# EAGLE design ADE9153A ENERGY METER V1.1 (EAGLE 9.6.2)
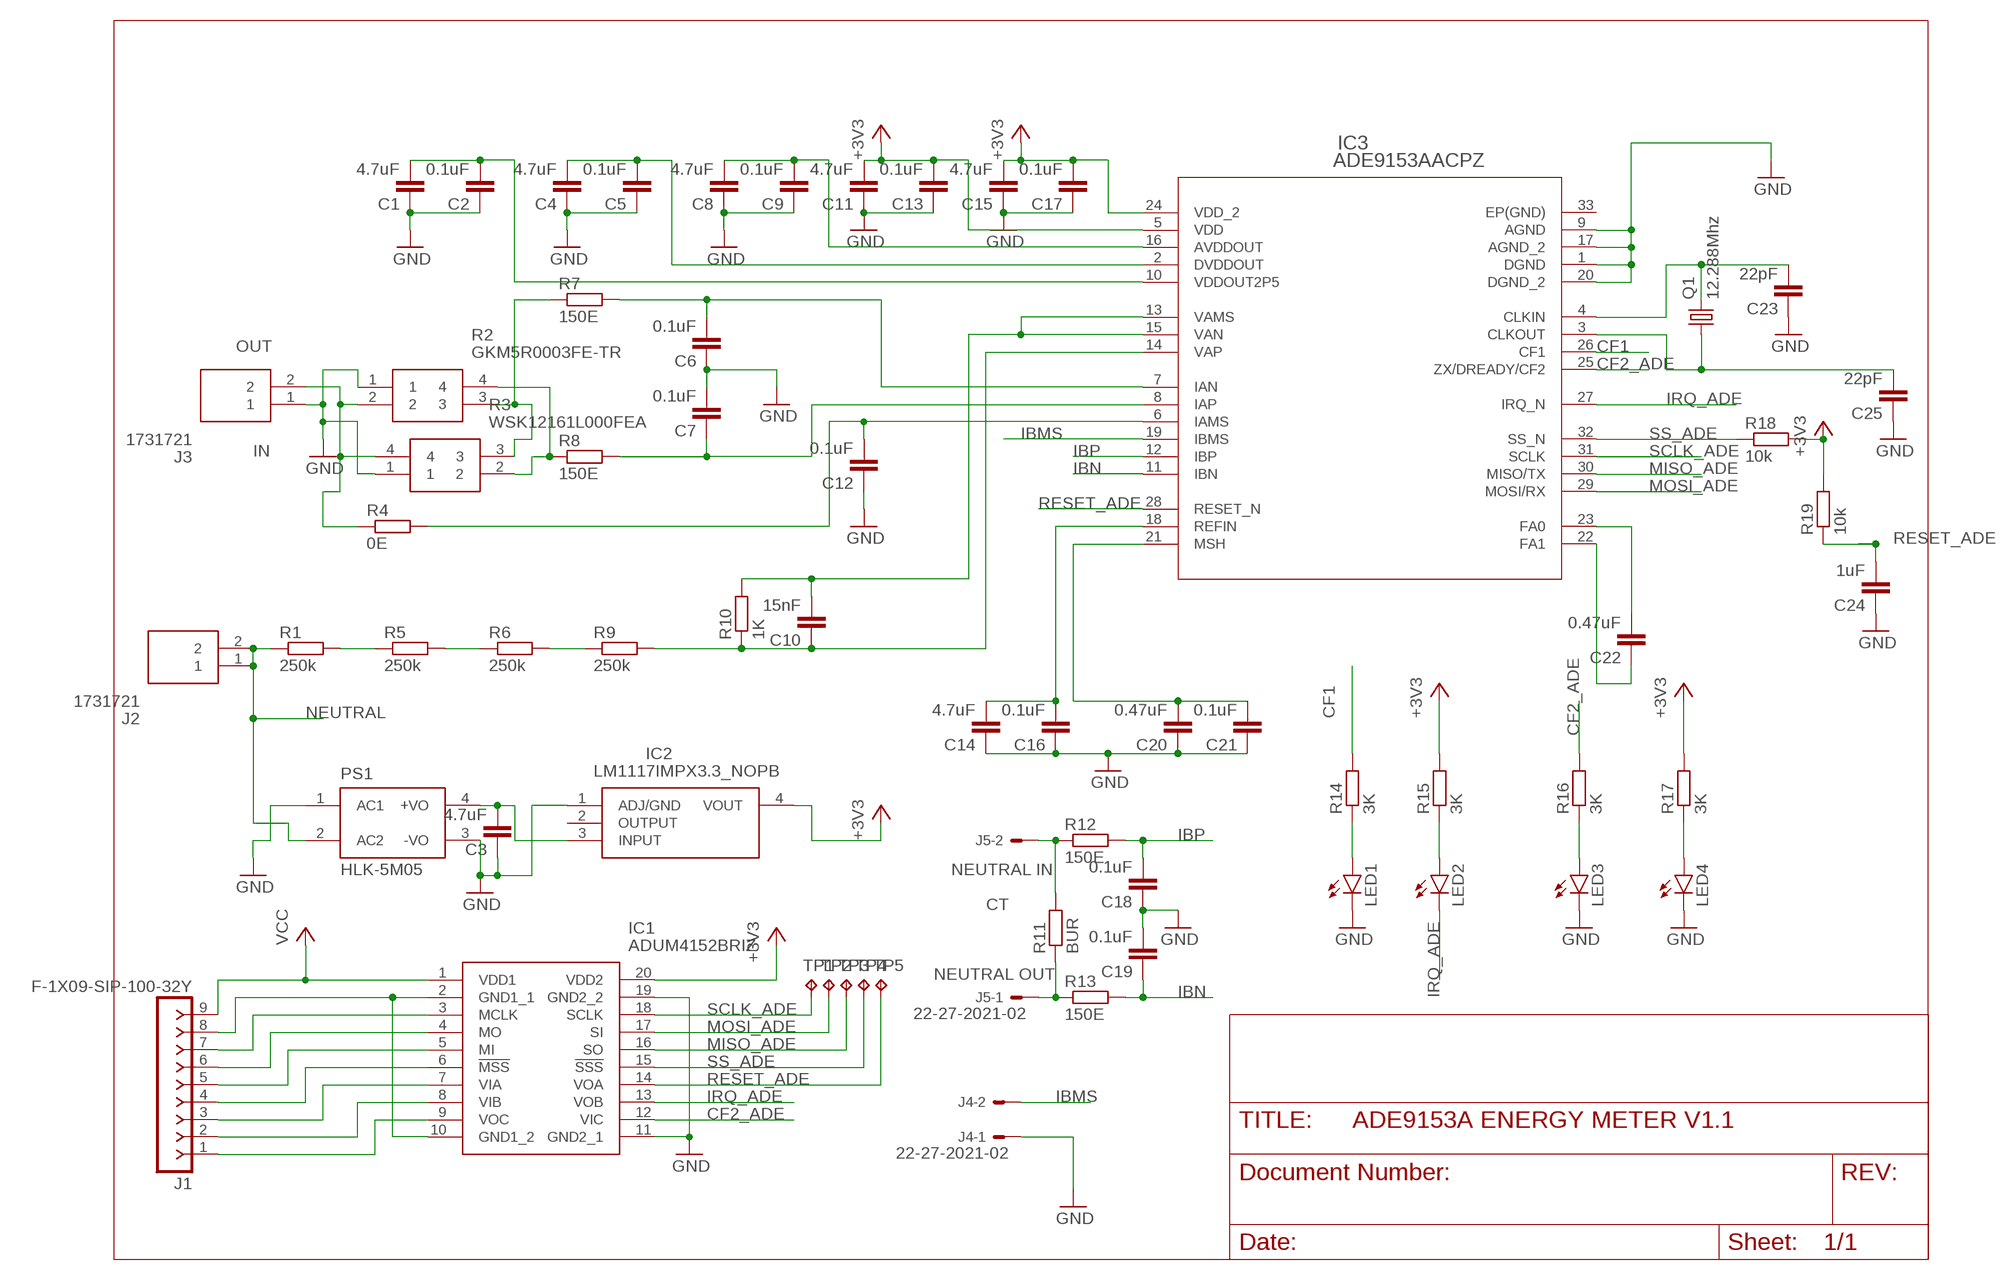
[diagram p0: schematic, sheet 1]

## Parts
C1  4.7uF  C-EUC0805K  [C0805K]
C2  0.1uF  C-EUC0805K  [C0805K]
C3  4.7uF  C-EUC0805K  [C0805K]
C4  4.7uF  C-EUC0805K  [C0805K]
C5  0.1uF  C-EUC0805K  [C0805K]
C6  0.1uF  C-EUC0805K  [C0805K]
C7  0.1uF  C-EUC0805K  [C0805K]
C8  4.7uF  C-EUC0805K  [C0805K]
C9  0.1uF  C-EUC0805K  [C0805K]
C10  15nF  C-EUC0805K  [C0805K]
C11  4.7uF  C-EUC0805K  [C0805K]
C12  0.1uF  C-EUC0805K  [C0805K]
C13  0.1uF  C-EUC0805K  [C0805K]
C14  4.7uF  C-EUC0805K  [C0805K]
C15  4.7uF  C-EUC0805K  [C0805K]
C16  0.1uF  C-EUC0805K  [C0805K]
C17  0.1uF  C-EUC0805K  [C0805K]
C18  0.1uF  C-EUC0805K  [C0805K]
C19  0.1uF  C-EUC0805K  [C0805K]
C20  0.47uF  C-EUC0805K  [C0805K]
C21  0.1uF  C-EUC0805K  [C0805K]
C22  0.47uF  C-EUC0805K  [C0805K]
C23  22pF  C-EUC0805K  [C0805K]
C24  1uF  C-EUC0805K  [C0805K]
C25  22pF  C-EUC0805K  [C0805K]
IC1  ADUM4152BRIZ  [SOIC127P1031X264-20N]
IC2  LM1117IMPX3.3_NOPB  [SOT230P700X180-4N]
IC3  ADE9153AACPZ  [QFN50P500X500X80-33N]
J1  F-1X09-SIP-100-32Y  [SIP-100-09-32Y]
J2  1731721  [1731721]
J3  1731721  [1731721]
J4  22-27-2021-02  [6410-02]
J5  22-27-2021-02  [6410-02]
LED1  LEDCHIPLED_1206  [CHIPLED_1206]
LED2  LEDCHIPLED_1206  [CHIPLED_1206]
LED3  LEDCHIPLED_1206  [CHIPLED_1206]
LED4  LEDCHIPLED_1206  [CHIPLED_1206]
PS1  HLK-5M05  [CONV_HLK-5M05]
Q1  12.288Mhz  CSM-7X-DU  [CSM-7X-DU]
R1  250k  R-EU_R0805  [R0805]
R2  GKM5R0003FE-TR  [GKM5R0003FETR]
R3  WSK12161L000FEA  [WSK12161L000FEA]
R4  0E  R-EU_R0805  [R0805]
R5  250k  R-EU_R0805  [R0805]
R6  250k  R-EU_R0805  [R0805]
R7  150E  R-EU_R0805  [R0805]
R8  150E  R-EU_R0805  [R0805]
R9  250k  R-EU_R0805  [R0805]
R10  1K  R-EU_R0805  [R0805]
R11  BUR  R-EU_R0805  [R0805]
R12  150E  R-EU_R0805  [R0805]
R13  150E  R-EU_R0805  [R0805]
R14  3K  R-EU_R0805  [R0805]
R15  3K  R-EU_R0805  [R0805]
R16  3K  R-EU_R0805  [R0805]
R17  3K  R-EU_R0805  [R0805]
R18  10k  R-EU_R0805  [R0805]
R19  10k  R-EU_R0805  [R0805]
TP1  TPTP10R  [TP10R]
TP2  TPTP10R  [TP10R]
TP3  TPTP10R  [TP10R]
TP4  TPTP10R  [TP10R]
TP5  TPTP10R  [TP10R]

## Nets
+3V3: C11.2 C13.2 C15.2 C17.2 IC1.20(VDD2) IC2.4(VOUT) IC3.5(VDD) IC3.24(VDD_2) R15.2 R17.2 R18.2 R19.2
CF1: IC3.26(CF1) R14.2
CF2_ADE: IC1.12(VIC) IC3.25(ZX/DREADY/CF2) R16.2
GND: C1.1 C2.1 C3.1 C4.1 C5.1 C6.1 C7.2 C8.1 C9.1 C11.1 C12.1 C13.1 C14.1 C15.1 C16.1 C17.1 C18.1 C19.2 C20.1 C21.1 C23.1 C24.1 C25.1 IC1.11(GND2_1) IC1.19(GND2_2) IC2.1(ADJ/GND) IC3.1(DGND) IC3.9(AGND) IC3.17(AGND_2) IC3.20(DGND_2) J3.1 J4.1 LED1.C LED3.C LED4.C PS1.1(AC1) PS1.3(-VO) R2.1 R3.1
IBMS: IC3.19(IBMS) J4.2
IBN: C19.1 IC3.11(IBN) R13.2
IBP: C18.2 IC3.12(IBP) R12.2
IRQ_ADE: IC1.13(VOB) IC3.27(IRQ_N) LED2.C
MISO_ADE: IC1.16(SO) IC3.30(MISO/TX) TP3.TP
MOSI_ADE: IC1.17(SI) IC3.29(MOSI/RX) TP2.TP
N$1: R2.4 R3.2 R8.1
N$2: R2.3 R3.3 R7.1
N$3: J5.2 R11.2 R12.1
N$4: C6.2 IC3.7(IAN) R7.2
N$5: C7.1 IC3.8(IAP) R8.2
N$6: C12.2 IC3.6(IAMS) R4.2
N$7: C3.2 IC2.3(INPUT) PS1.4(+VO)
N$8: R1.2 R5.1
N$9: R5.2 R6.1
N$10: R6.2 R9.1
N$11: C10.1 IC3.14(VAP) R9.2 R10.1
N$12: C10.2 IC3.13(VAMS) IC3.15(VAN) R10.2
N$13: C8.2 C9.2 IC3.16(AVDDOUT)
N$14: C14.2 C16.2 IC3.18(REFIN)
N$15: LED1.A R14.1
N$16: LED2.A R15.1
N$17: C1.2 C2.2 IC3.10(VDDOUT2P5)
N$18: C4.2 C5.2 IC3.2(DVDDOUT)
N$19: C23.2 IC3.4(CLKIN) Q1.2
N$20: C25.2 IC3.3(CLKOUT) Q1.1
N$22: C22.2 IC3.23(FA0)
N$23: C22.1 IC3.22(FA1)
N$24: IC1.2(GND1_1) IC1.10(GND1_2) J1.8
N$25: C20.2 C21.2 IC3.21(MSH)
N$26: IC1.3(MCLK) J1.7
N$27: IC1.4(MO) J1.6
N$28: IC1.5(MI) J1.5
N$29: IC1.6(!MSS) J1.4
N$30: IC1.7(VIA) J1.3
N$31: IC1.8(VIB) J1.2
N$32: IC1.9(VOC) J1.1
N$33: LED3.A R16.1
N$34: LED4.A R17.1
N$35: J5.1 R11.1 R13.1
N$38: J3.2 R2.2 R3.4 R4.1
NEUTRAL: J2.1 J2.2 PS1.2(AC2) R1.1
RESET_ADE: C24.2 IC1.14(VOA) IC3.28(RESET_N) R19.1 TP5.TP
SCLK_ADE: IC1.18(SCLK) IC3.31(SCLK) TP1.TP
SS_ADE: IC1.15(!SSS) IC3.32(SS_N) R18.1 TP4.TP
VCC: IC1.1(VDD1) J1.9
Unconnected: IC2.2(OUTPUT) IC3.33(EP(GND))

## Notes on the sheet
- OUT
- IN
- NEUTRAL IN
- CT
- NEUTRAL OUT

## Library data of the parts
C1-C25 = rcl:C-EU: CAPACITOR, European symbol; SPICEPREFIX: C
IC1 = IC:ADUM4152BRIZ: Analog Devices ADUM4152BRIZ PCB SMT, 7-channel Digital Isolator for SPI 34MBps, 5 kV ac, 20-Pin SOIC Source: Datasheet; ARROW_PART_NUMBER: ADUM4152BRIZ; ARROW_PRICE-STOCK: https://www.arrow.com/en/products/adum4152briz/analog-devices; DESCRIPTION: Analog Devices ADUM4152BRIZ PCB SMT, 7-channel Digital Isolator for SPI 34MBps, 5 kV ac, 20-Pin SOIC; HEIGHT: 2.64mm; MANUFACTURER_NAME: Analog Devices; MANUFACTURER_PART_NUMBER: ADUM4152BRIZ; MOUSER_PART_NUMBER: 584-ADUM4152BRIZ; MOUSER_PRICE-STOCK: https://www.mouser.co.uk/ProductDetail/Analog-Devices/ADUM4152BRIZ/?qs=iCT64eccu7h2dAwNIWQgpQ%3D%3D
IC2 = IC:LM1117IMPX3.3_NOPB: Space Saving 800mA Low-Dropout Linear Regulator with Internal Current Limit 4-SOT-223 -40 to 125 Source: Datasheet; DESCRIPTION: Space Saving 800mA Low-Dropout Linear Regulator with Internal Current Limit 4-SOT-223 -40 to 125; HEIGHT: 1.8mm; MANUFACTURER_NAME: Texas Instruments; MANUFACTURER_PART_NUMBER: LM1117IMPX3.3/NOPB
IC3 = ADE9153AACPZ:ADE9153AACPZ; AVAILABILITY: Unavailable; DESCRIPTION: Single Phase Meter IC 32-LFCSP (5x5); MF: Analog Devices; MP: ADE9153AACPZ; PACKAGE: LFCSP -32 Analog Devices; PRICE: None
J1 = con-headers-jp:F-1X09-: FEMALE HEADER
J2 J3 = IC:1731721: 2 way PCB mount screw terminal,7.62mm 2 way PCB mount screw terminal,7.62mm; ARROW_PART_NUMBER: 1731721; ARROW_PRICE-STOCK: https://www.arrow.com/en/products/1731721/phoenix-contact; DESCRIPTION: 2 way PCB mount screw terminal,7.62mm 2 way PCB mount screw terminal,7.62mm; HEIGHT: mm; MANUFACTURER_NAME: Phoenix Contact; MANUFACTURER_PART_NUMBER: 1731721; MOUSER_PART_NUMBER: 651-1731721; MOUSER_PRICE-STOCK: https://www.mouser.co.uk/ProductDetail/Phoenix-Contact/1731721?qs=Hp4IEBVVqKLHS2iTGzgL4g%3D%3D
J4 J5 = con-molex:22-?-02: CONNECTOR; MF: MOLEX; OC_FARNELL: unknown; OC_NEWARK: unknown
LED1-LED4 = led:LED: LED
PS1 = HLK-5M05:HLK-5M05: AC DC 220V to 5V 5W 5Watt Isolated Switching Step-Down Power Supply Module Converter; AVAILABILITY: Unavailable; MF: Hi-link; MP: HLK-5M05; PACKAGE: Package; PRICE: None
Q1 = crystal:CSM-7X-DU: SMD CRYSTAL; OC_FARNELL: unknown; OC_NEWARK: unknown
R1 R4-R19 = rcl:R-EU_: RESISTOR, European symbol; SPICEPREFIX: R
R2 = IC:GKM5R0003FE-TR: FK/GK Series Metal Alloy Low-Resistance Chip Resistor Source: Datasheet; DESCRIPTION: FK/GK Series Metal Alloy Low-Resistance Chip Resistor; HEIGHT: 3.5mm; MANUFACTURER_NAME: Ohmite; MANUFACTURER_PART_NUMBER: GKM5R0003FE-TR; MOUSER_PART_NUMBER: 588-GKM5R0003FE-TR; MOUSER_PRICE-STOCK: https://www.mouser.co.uk/ProductDetail/Ohmite/GKM5R0003FE-TR/?qs=0lSvoLzn4L%252BprfgVSUIuyQ%3D%3D
R3 = WSK12161L000FEA:WSK12161L000FEA: Check prices; AVAILABILITY: Warning; DESCRIPTION: 1 mOhms ±1% 3W Chip Resistor Wide 1612 (3831 Metric), 1216 Current Sense, Moisture Resistant, Pulse Withstanding Metal Element; MF: Vishay Dale; MP: WSK12161L000FEA; PACKAGE: 1216 Vishay Dale; PRICE: None; PURCHASE-URL: https://pricing.snapeda.com/search/part/WSK12161L000FEA/?ref=eda
TP1-TP5 = testpad:TP: Test pad

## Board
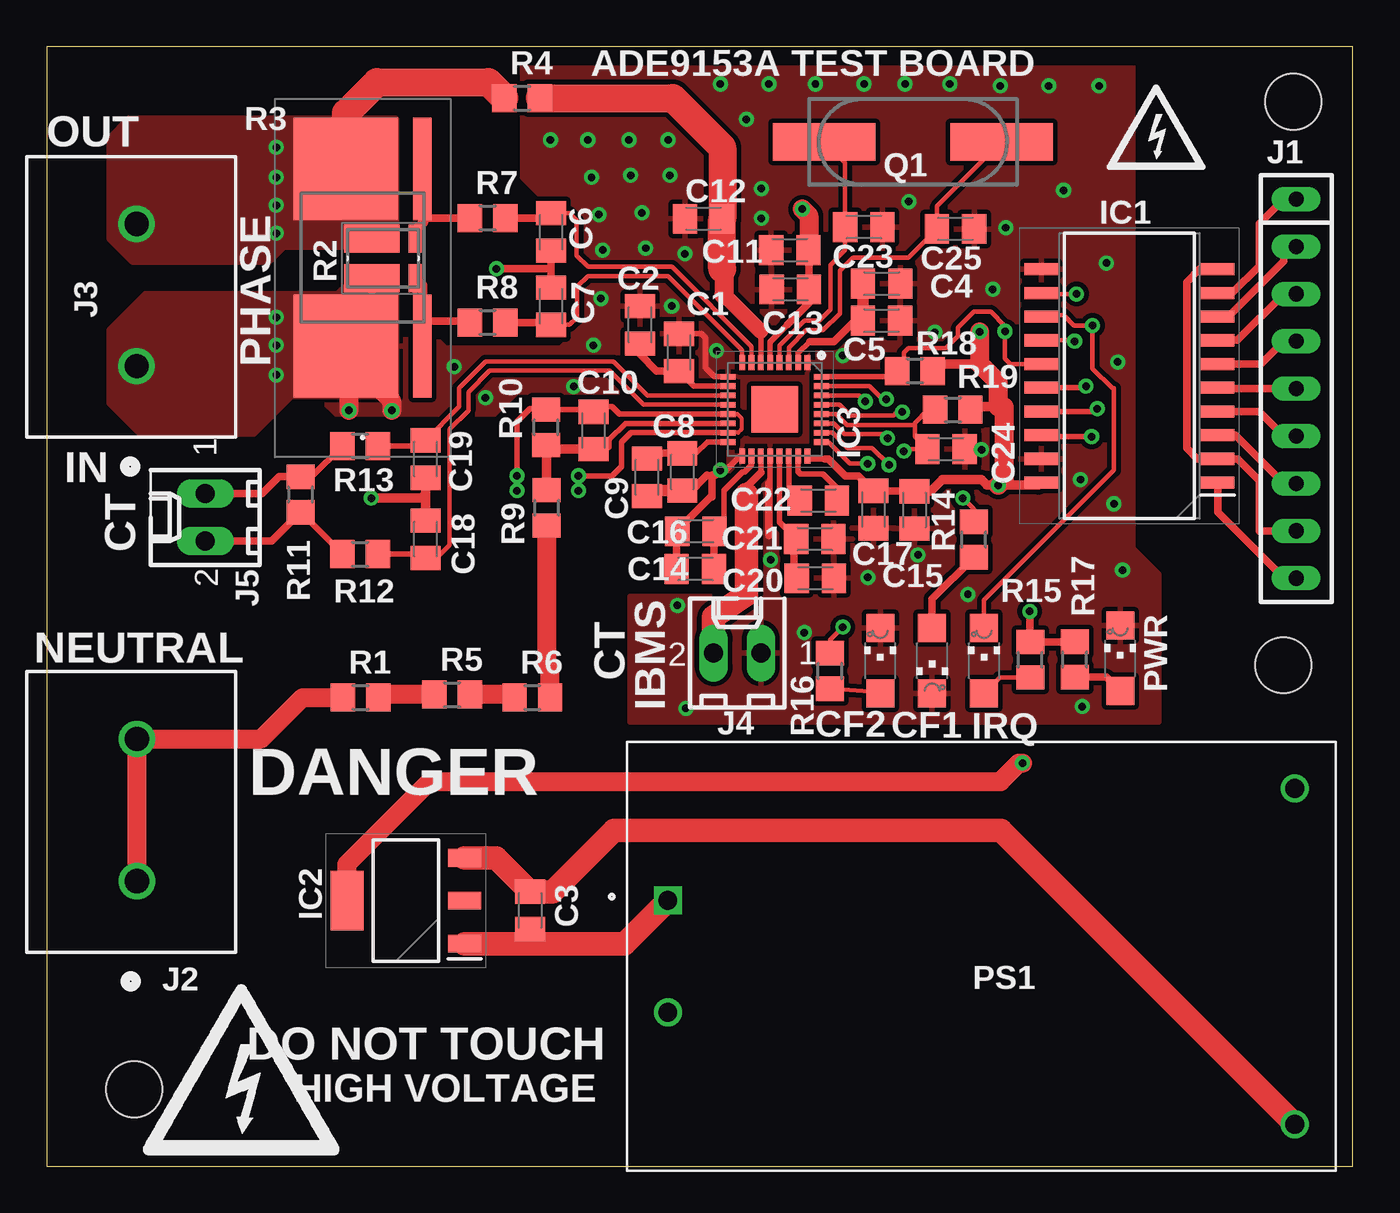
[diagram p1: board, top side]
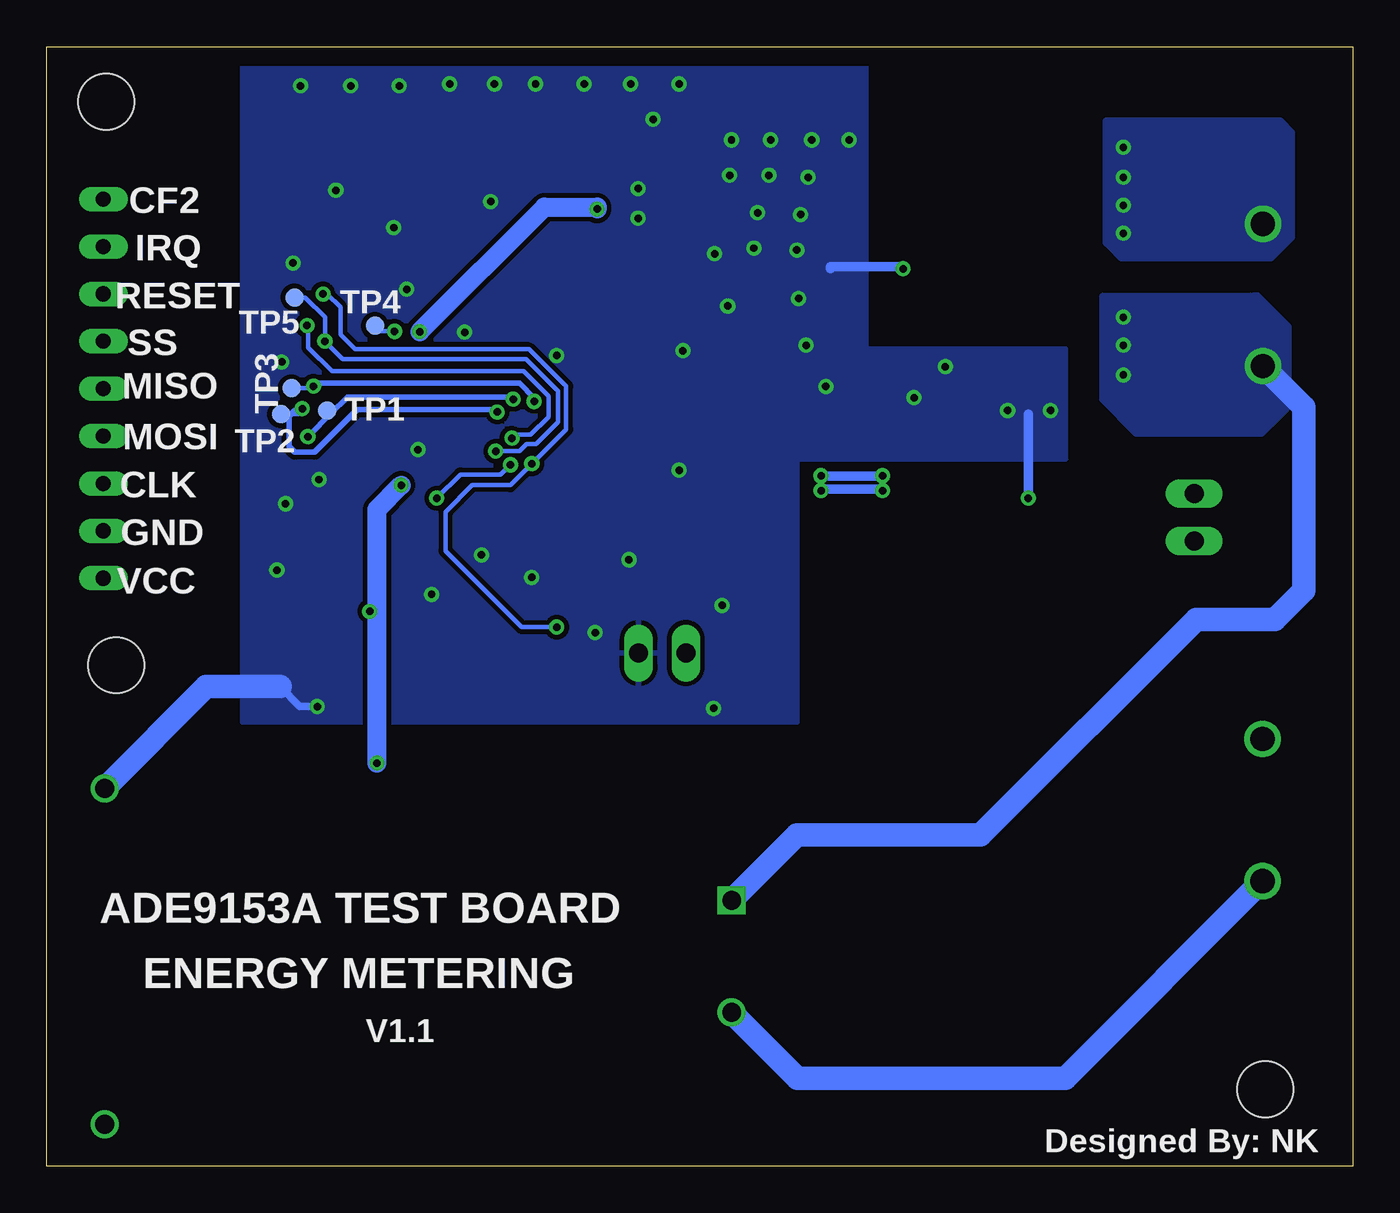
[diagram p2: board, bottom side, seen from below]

Size 70 x 60 mm. Coordinates in mm from the lower left corner, seen from the top.
Outline: 0,0 70,0 70,60 0,60 0,0
Copper layers (1*16): Top 0.035mm / dielectric 1.5mm / Bottom 0.035mm
Design rules "default": minimum track width 6mil, minimum drill 0.35mm, track to track 6mil, track to pad 6mil, pad to pad 6mil, via to via 6mil, smd to smd 6mil, copper to edge 40mil, drill to drill 6mil, minimum pad ring 10mil, minimum via ring 8mil, stop-mask expansion 4mil, vias tented up to drill 0mil, thermal gap 10mil
Holes 3 mm at 4.69,4.13 66.8,57.04 66.27,26.85

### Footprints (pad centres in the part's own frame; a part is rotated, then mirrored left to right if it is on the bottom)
C0805K = smd 1.3 x 1.6: 1 -1,0; 2 1,0
SOIC127P1031X264-20N = smd 1.8 x 0.65: 1 -4.725,5.715; 2 -4.725,4.445; 3 -4.725,3.175; 4 -4.725,1.905; 5 -4.725,0.635; 6 -4.725,-0.635; 7 -4.725,-1.905; 8 -4.725,-3.175; 9 -4.725,-4.445; 10 -4.725,-5.715; 11 4.725,-5.715; 12 4.725,-4.445; 13 4.725,-3.175; 14 4.725,-1.905; 15 4.725,-0.635; 16 4.725,0.635; 17 4.725,1.905; 18 4.725,3.175; 19 4.725,4.445; 20 4.725,5.715
SOT230P700X180-4N = smd 1.75 x 0.95: 1 -3.15,2.3; 2 -3.15,0; 3 -3.15,-2.3 | smd 1.75 x 3.2: 4 3.15,0
QFN50P500X500X80-33N = smd 0.8 x 0.3: 1 -2.5,1.75; 2 -2.5,1.25; 3 -2.5,0.75; 4 -2.5,0.25; 5 -2.5,-0.25; 6 -2.5,-0.75; 7 -2.5,-1.25; 8 -2.5,-1.75; 17 2.5,-1.75; 18 2.5,-1.25; 19 2.5,-0.75; 20 2.5,-0.25; 21 2.5,0.25; 22 2.5,0.75; 23 2.5,1.25; 24 2.5,1.75 | smd 0.3 x 0.8: 9 -1.75,-2.5; 10 -1.25,-2.5; 11 -0.75,-2.5; 12 -0.25,-2.5; 13 0.25,-2.5; 14 0.75,-2.5; 15 1.25,-2.5; 16 1.75,-2.5; 25 1.75,2.5; 26 1.25,2.5; 27 0.75,2.5; 28 0.25,2.5; 29 -0.25,2.5; 30 -0.75,2.5; 31 -1.25,2.5; 32 -1.75,2.5 | smd 2.5 x 2.5: 33 0,0
SIP-100-09-32Y = drill 0.813 long: 1 -10.16,0; 2 -7.62,0; 3 -5.08,0; 4 -2.54,0; 5 0,0; 6 2.54,0; 7 5.08,0; 8 7.62,0; 9 10.16,0
1731721 = drill 1.3 pad 1.95: 1 -3.92,-0.11; 2 3.7,-0.11
6410-02 = drill 1.016 long: 1 1.27,0; 2 -1.27,0
CHIPLED_1206 = smd 1.5 x 1.5: A 0,-1.75; C 0,1.75
CONV_HLK-5M05 = drill 1 pad 1.5 square: 1 -16.8,3 | drill 1 pad 1.5: 2 -16.8,-3; 3 16.8,9; 4 16.8,-9
CSM-7X-DU = smd 5.5 x 2: 1 -4.75,0; 2 4.75,0
R0805 = smd 1.3 x 1.5: 1 -0.95,0; 2 0.95,0
GKM5R0003FETR = smd 5.5 x 5.6: 1 -4.75,0.9; 2 4.75,0.9 | smd 5.5 x 1: 3 4.75,-3.2; 4 -4.75,-3.2
WSK12161L000FEA = smd 2.95 x 1.495: 1 -0.6,-1.053; 4 -0.6,1.053 | smd 0.7 x 1.495: 2 1.725,-1.053; 3 1.725,1.053
TP10R = smd 1 x 1: TP 0,0

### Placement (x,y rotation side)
C1  33.89,43.61 270 top
C2  31.79,45.09 270 top
C3  25.91,13.71 90 top
C4  44.75,47.29 180 top
C5  44.74,45.31 180 top
C6  27.03,50.07 90 top
C7  27.03,46.09 90 top
C8  34.06,37.21 90 top
C9  32.17,36.92 90 top
C10  29.31,39.43 90 top
C11  39.83,49.09 0 top
C12  35.21,50.77 0 top
C13  39.85,46.99 0 top
C14  34.76,32.01 0 top
C15  46.51,35.17 90 top
C16  34.79,34.03 0 top
C17  44.31,35.19 90 top
C18  20.3,33.6 270 top
C19  20.3,37.9 270 top
C20  41.19,31.51 180 top
C21  41.17,33.61 180 top
C22  41.35,35.67 0 top
C23  43.79,50.33 180 top
C24  48.2,38.43 180 top
C25  48.71,50.23 180 top
IC1  58.02,42.35 180 top
IC2  19.25,14.23 180 top
IC3  39.02,40.56 270 top
J1  66.96,41.67 270 top
J2  4.73,19.2 90 top
J3  4.71,46.8 90 top
J4  37.01,27.5 0 top
J5  8.5,34.77 90 top
LED1  47.45,27.09 180 top
LED2  50.23,27.09 0 top
LED3  44.67,27.09 0 top
LED4  57.53,27.22 0 top
PS1  50.09,11.25 0 top
Q1  46.42,54.9 180 top
R1  16.83,25.12 0 top
R2  16.94,48.7 90 top
R3  18.03,48.65 0 top
R4  25.48,57.24 0 top
R5  21.73,25.27 0 top
R6  26.03,25.12 0 top
R7  23.63,50.82 0 top
R8  23.63,45.22 0 top
R9  26.8,35.29 90 top
R10  26.76,39.6 90 top
R11  13.6,36 270 top
R12  16.8,32.8 0 top
R13  16.8,38.6 0 top
R14  49.68,33.58 90 top
R15  52.71,27.14 90 top
R16  41.98,26.54 90 top
R17  55.09,27.16 90 top
R18  46.53,42.62 0 top
R19  48.56,40.54 0 top
TP1  54.97,40.5 0 bottom
TP2  57.44,40.3 0 bottom
TP3  56.88,41.69 0 bottom
TP4  52.4,45.05 0 bottom
TP5  56.72,46.56 0 bottom

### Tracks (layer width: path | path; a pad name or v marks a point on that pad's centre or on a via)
+3V3  (via drill 0.4)
  Top 0.305: IC3.5 38.77,44.17 39.7,45.1 | 40.85,49.07 C11.2 | IC3.24 40.93,37.9 41.7,37.9
  Top 0.406: 39.7,45.1 40.85,46.25 C13.2 40.85,49.07 | 41.7,37.9 41.9,37.9 42.8,37 43.5,37 C17.2 46.49,36.19 C15.2 | R17.2 55.09,28.36 54.83,28.09 R15.2 52.69,28.21 v52.69,29.73
  Top 0.508: R18.2 47.86,43 50,43 | R19.2 49.67,40.7 51,40.7 51.3,40.7 | IC1.20 53.16,36.5 v51,36.5 50.4,36.5 50.1,36.8 48,36.8 47.39,36.19 46.49,36.19
  Top 1.016: IC2.4 16.1,16.2 20.52,20.62 51.12,20.62 52.1,21.6 v52.3,21.6 | v51,36.5 51.3,36.8 51.3,40.7 | 51,40.7 51,42 50.01,42.99 | 50.01,42.99 50,43 | 50.01,42.99 v50.01,44.72 | v40.5,51.3 40.85,50.95 40.85,49.07
  Bottom 0.406: v52.69,29.73 52.3,30.12
  Bottom 1.016: v52.3,21.6 52.3,30.12 52.3,35.2 v51,36.5 | v50.01,44.72 43.33,51.4 40.5,51.4 v40.5,51.3
CF1  (via drill 0.4)
  Top 0.254: IC3.26 42.12,39.31 42.92,38.5 44.24,38.5 v45.15,37.59 | v49.1,35.8 49.68,35.22 R14.2
  Bottom 0.254: v45.15,37.59 45.67,37.07 47.83,37.07 v49.1,35.8
CF2_ADE  (via drill 0.4)
  Top 0.254: IC3.25 41.89,38.81 43.05,37.65 v44,37.65 | v42.67,28.89 41.98,28.2 R16.2 | v55.19,46.74 53.36,46.74 IC1.12
  Bottom 0.254: v42.67,28.89 44.54,28.89 48.63,32.98 48.63,35.07 47.2,36.5 45.15,36.5 v44,37.65 42.16,39.49 42.16,41.8 44.15,43.79 53.47,43.79 54.25,44.57 54.25,46.03 54.96,46.74 v55.19,46.74
GND  (via drill 0.4)
  Top 0.254: 38.77,36.67 38.7,36.6
  Top 0.305: IC3.20 38.77,36.67 | IC3.17 37.16,38.06 36.14,37.04 35.66,37.04 35.65,37.04 35.4,37.04 | 34.31,35.95 C8.1 | IC3.9 35.79,42.31 35.3,42.8 35.3,44.4 35.09,44.61 C1.1
  Top 0.406: C7.2 27.03,48.1 | 27.03,48.1 C6.1 | 27.03,48.1 v24.1,48.1 | 34.31,35.95 35.4,37.04 | R3.1 17.43,45.02 16.2,43.79 | 38.7,36.6 38.7,33.8 | 35.66,37.04 35.66,35.85 35.58,35.85 33.79,34.06 | C16.1 33.79,34.06 | v36.1,37.3 35.84,37.04 35.65,37.04 | C14.1 33.76,34.03 33.79,34.06
  Top 0.508: C18.1 20.3,36 | 20.3,36 C19.2 | 20.3,36 20.1,35.8 v17.4,35.8 | C24.1 50.07,38.43 v50.1,38.4
  Top 0.61: C8.1 32.46,36.21 C9.1
  Top 1.016: v16.2,40.5 16.2,43.79 R2.1 16.04,43.46 18.5,41 v18.5,40.5
  Top 1.27: IC2.1 26.1,11.93 | C3.1 26.1,12.52 26.1,11.93 | PS1.1 30.97,11.93 26.1,11.93
  Bottom 0.406: v55.5,24.63 56.43,24.63 57.5,25.7
  Bottom 0.508: v24.1,48.1 24.2,48.2 28,48.2 28,48.1 | v17.4,35.8 17.4,40.3
  Bottom 1.27: PS1.3 61.44,25.7 57.5,25.7 | J3.1 2.62,40.68 2.62,30.86 4.18,29.3 8.4,29.3 19.95,17.75 29.79,17.75 PS1.1
  other vias: 27,55 29,55 31.2,55 33.3,55 33.4,53.1 31.3,53.1 29.2,53 29.6,51 31.9,51.1 29.8,49.1 34.2,48.9 32.1,49.2 29.7,46.5 29.3,44 21.84,42.85 12.3,45.5 12.3,44 12.3,42.4 35.9,43.7 42.67,43.45 40.6,28.6 44.01,31.56 46.7,32.76 49.37,30.64 57.66,31.94 55.4,36.8 57.2,35.5 57.4,43.1 50.7,47 47.6,44.7 54.5,52.3 56.4,57.9 38.7,58 36.1,58 41.2,58 43.8,58 46,58 48.4,58 51.1,57.9 53.7,57.9 37.5,56.1 38.3,52.4 46.2,51.7 51.4,50.3 56.8,48.4 38.3,50.8 33.5,46.1 34.26,24.54 38.8,32.5 23.52,41.18 28.24,41.79 33.8,30.06
  pour Top (isolate 0.254): 25.5,59.2 25.5,53 28.2,50.3 28.2,44.5 27.55,43.85 21.35,43.85 20.9,44.3 15.6,44.3 14.8,43.5 14.8,41 15.5,40.3 24,40.3 25.2,41.5 35.4,41.5 36.58,40.32 36.58,30.52 31.26,30.52 31.26,23.82 59.6,23.82 59.6,31.7 58.2,33.1 58.2,60.8 25.5,60.8 25.5,59.3 25.6,59.2
  pour Bottom (isolate 0.254): 15.4,37.9 29.8,37.9 29.8,23.8 59.5,23.8 59.5,60.7 26.4,60.7 26.1,60.4 26.1,43.8 15.4,43.8
  pour Top (no thermals): 16.2,47.9 16.2,47.3 15.6,46.7 5.3,46.7 3.4,44.8 3.4,40.9 5,39.3 11.1,39.3 13.1,41.3 18.6,41.3 18.7,41.4 18.7,47.9
  pour Bottom (no thermals): 5.2,46.7 3.5,45 3.5,40.7 4.9,39.3 11.6,39.3 13.4,41.1 13.4,46.6 5.3,46.6
IBMS
  Top 0.305: IC3.19 38.27,37.17
  Top 0.406: 38.27,37.17 37.5,36.4
  Top 0.508: 37.5,36.4 37.5,36
  Top 1.27: 37.5,36 37.5,30.63 35.74,29.42 J4.2
IBN
  Top 0.254: C19.1 22.1,40.7 22.1,41.7 23.51,43.11 30.39,43.11 32.19,41.31 IC3.11
  Top 0.305: C19.1 20,38.6 R13.2
IBP
  Top 0.254: IC3.12 31.99,40.81 30.17,42.63 23.73,42.63 22.6,41.5 22.6,40.5 21.6,39.5 21.6,33.3 20.9,32.6 C18.2
  Top 0.305: R12.2 20.1,32.8 C18.2
IRQ_ADE  (via drill 0.4)
  Top 0.254: IC3.27 42.19,39.81 42.76,39.24 44.76,39.24 44.98,39.02 v45.06,39.02 | IC1.13 53.37,45.6 54.5,45.6 55.04,45.06 v56.04,45.06 56.04,42.76 57.1,41.7 57.2,41.7 57.2,37.3 50.23,30.33 LED2.C
  Bottom 0.254: v45.06,39.02 44.87,39.21 44.06,39.21 43.11,40.16 43.11,41.27 44.44,42.6 54.7,42.6 55.98,43.88 55.98,44.99 v56.04,45.06
MISO_ADE  (via drill 0.4)
  Top 0.254: IC3.30 43.55,41.31 v43.87,40.99
  Top 0.305: v55.7,41.8 55.62,41.72 IC1.16
  Bottom 0.254: TP3.TP 55.81,41.69 v55.7,41.8
  Bottom 0.305: v43.87,40.99 43.87,41.17 44.66,41.96 55.54,41.96 v55.7,41.8
MOSI_ADE  (via drill 0.4)
  Top 0.254: IC3.29 42.49,40.81 43.07,40.23 45.38,40.23 45.57,40.42 v45.85,40.42
  Top 0.305: v56.3,40.6 56.15,40.45 IC1.17
  Bottom 0.254: TP2.TP 56.5,40.3 56.3,40.5
  Bottom 0.305: v45.85,40.42 45.98,40.55 53.35,40.55 55.63,38.27 56.7,38.27 57,38.57 57,40.2 56.7,40.5 56.3,40.5 v56.3,40.6
N$1
  Top 0.254: 20.53,45.3 19.75,46.08 R3.2 | 22.68,45.3 R8.1
  Top 0.406: 20.53,45.3 22.68,45.3
  Top 0.508: R2.4 20.14,47.21 R3.2
N$2
  Top 0.254: R2.3 20.14,50.8 | 22.66,50.8 R7.1
  Top 0.406: 20.14,50.8 22.66,50.8
  Top 0.508: R3.3 19.75,50.16 20.2,50.6 20.2,53.39 R2.3
N$3
  Top 0.305: R12.1 R11.2
  Top 0.406: J5.2 12.05,33.5 R11.2
N$4
  Top 0.254: 26.91,50.95 C6.2 | 26.78,50.82 C6.2 | C6.2 28.03,51.07 28.4,50.7 28.4,48.8 29,48.2 33.5,48.2 37.77,43.93 IC3.7
  Top 0.406: R7.2 26.78,50.82
N$5
  Top 0.254: 26.9,45.22 C7.1 28.03,45.09 28.43,45.49 28.43,47.13 29,47.7 33.3,47.7 37.27,43.73 IC3.8
  Top 0.406: R8.2 26.9,45.22
N$6
  Top 0.305: IC3.6 38.27,44.73
  Top 0.813: 38.27,44.73 36.3,46.7
  Top 1.016: 36.2,48.1 36.3,48 36.3,46.7
  Top 1.5: R4.2 33.56,57.24 36.21,54.59 C12.2 36.2,50.76 36.2,48.1
N$7
  Top 1.27: IC2.3 24.09,16.53 C3.2 27.12,14.71 30.41,18 51.14,18 PS1.4
N$8
  Top 1.016: R1.2 17.93,25.27 R5.1
N$9
  Top 1.016: R5.2 24.93,25.27 R6.1
N$10
  Top 1.016: R9.1 26.8,27 26.98,26.82 R6.2
N$11
  Top 0.305: IC3.14 31.01,39.81 30.13,38.93 30.13,38.55 30.01,38.43 C10.1
  Top 0.508: R9.2 26.8,38.61 | 26.8,38.61 R10.1 | C10.1 26.98,38.43 26.8,38.61
N$12  (via drill 0.4)
  Top 0.203: IC3.13 37.02,40.31 37.23,40.1 37.23,39.49 37.05,39.31 IC3.15
  Top 0.305: IC3.15 31.31,39.31 30.8,38.8 30.8,37.5 30.3,37 28.6,37 | v28.5,36.2 28.5,36.9 28.6,37 | 28.6,37 v28.5,37 | 29.19,40.55 R10.2 26.71,40.6 25.9,40.6 25.2,39.9 v25.2,37 v25.2,36.2 | 29.19,40.55 C10.2 | IC3.13 30.69,40.31 30.3,40.7 29.34,40.7 29.19,40.55
  Bottom 0.305: v28.5,37 v28.5,36.2 | v25.2,36.2 v25.2,37
  Bottom 0.508: v28.5,37 v25.2,37 | v28.5,36.2 28.4,36.3 25.3,36.3 v25.2,36.2
N$13
  Top 0.305: IC3.16 35.41,38.81 34.81,38.21 C8.2
  Top 0.406: C9.2 32.46,38.21 C8.2
N$14
  Top 0.305: IC3.18 37.77,37.57 37.4,37.2 37.3,37.2 36.3,36.2 36.3,34.54 C16.2 35.76,34
  Top 0.406: 35.76,34 C14.2
N$15
  Top 0.406: R14.1 47.45,30.4 LED1.A
N$16
  Top 0.254: LED2.A 51.08,26.19 R15.1
N$17
  Top 0.305: IC3.10 34.69,41.81 C1.2
  Top 0.406: C1.2 32.69,42.61 31.79,43.51 C2.2
N$18
  Top 0.305: IC3.2 40.27,43.56 40.91,44.2
  Top 0.406: 40.91,44.2 42.2,44.2 43.31,45.31 C5.2
  Top 0.61: C5.2 C4.2
N$19
  Top 0.254: Q1.2 42.79,53.78 C23.2 42.79,49.09 42,48.3 42,45.9 41.42,45.32 40.6,45.32 39.27,43.99 IC3.4
N$20
  Top 0.254: IC3.3 39.77,43.87 40.7,44.8 41.6,44.8 42.5,45.7 42.5,48 43.2,48.7 46.18,48.7 C25.2 47.71,51.44 Q1.1
N$22
  Top 0.305: IC3.23 40.27,37.23 40.4,37.1 41.6,37.1 42.35,36.35 C22.2
N$23
  Top 0.305: IC3.22 39.77,36.45 40.35,35.87 C22.1
N$24
  Top 0.406: J1.8 65,34.05 65,36.73 63.83,37.91 IC1.2 61.67,37.91 61.09,38.49 61.09,47.39 61.77,48.07 IC1.10
N$25
  Top 0.305: C21.2 40.04,33.74 39.27,34.51 IC3.21
  Top 0.406: C20.2 40.04,31.66 40.04,33.74
N$26
  Top 0.406: J1.7 66.3,36.59 63.71,39.18 IC1.3
N$27
  Top 0.406: J1.6 66.3,39.13 64.98,40.45 IC1.4
N$28
  Top 0.406: J1.5 66.3,41.67 62.8,41.67 IC1.5
N$29
  Top 0.406: J1.4 66.3,44.21 65.08,42.99 IC1.6
N$30
  Top 0.406: J1.3 66.3,46.75 63.81,44.26 IC1.7
N$31
  Top 0.406: J1.2 66.3,49.29 66.3,48.51 63.33,45.53 IC1.8
N$32
  Top 0.406: J1.1 66.3,51.83 64.97,50.51 64.97,48.25 63.52,46.8 IC1.9
N$33
  Top 0.254: R16.1 44.8,25.39 LED3.A
N$34
  Top 0.406: LED4.A 56.79,26.21 R17.1
N$35
  Top 0.305: R11.1 14.2,36.95 R13.1
  Top 0.406: J5.1 11.54,36.04 12.45,36.95 R11.1
N$38  (via drill 0.4)
  Top 1.5: R2.2 16.04,56.44 17.7,58.1 23.67,58.1 R4.1
  other vias: 12.3,54.6 12.3,53 12.3,51.5 12.3,50
  pour Top (no thermals): 3.4,55.1 3.4,49.7 4.6,48.5 11.9,48.5 12.7,49.3 18.7,49.3 18.7,56.1 4.4,56.1
  pour Bottom (no thermals): 3.3,55.3 3.3,49.8 4.4,48.7 12.4,48.7 13,49.3 13.2,49.5 13.2,56 3.9,56 3.3,55.4
NEUTRAL
  Top 1.016: J2.1 J2.2 11.5,22.9 13.72,25.12 R1.1
  Bottom 1.27: J2.1 15.4,4.72 29.76,4.72 PS1.2
RESET_ADE  (via drill 0.4)
  Top 0.254: IC1.14 55.02,44.26 55.07,44.21 v55.09,44.21 | v45.93,38.32 46.04,38.43 C24.2 | C24.2 47.61,38.84 | IC3.28 42.29,40.31 42.89,39.71 46.52,39.71 | R19.1 47.23,40.54 46.52,39.83 46.52,39.71 | 46.52,39.71 46.52,39.47 46.54,39.47 46.54,39.09 C24.2
  Bottom 0.254: v45.93,38.32 44.66,38.32 44.27,38.71 43.78,38.71 42.6,39.89 42.6,41.55 44.3,43.25 54.13,43.25 v55.09,44.21 v55.08,44.22 55.08,45.49 56.15,46.56 TP5.TP
SCLK_ADE  (via drill 0.4)
  Top 0.254: IC3.31 44.09,41.81 44.9,41
  Top 0.305: 44.9,41 v45,41.1 | v56,39.1 53.38,39.1 IC1.18
  Bottom 0.254: TP1.TP 54.82,40.35 54.74,40.35
  Bottom 0.305: v45,41.1 45.13,41.23 53.87,41.23 54.74,40.35 v56,39.1
SS_ADE  (via drill 0.4)
  Top 0.254: R18.1 45.93,42.97 45.93,43.6 46.17,43.84 48.2,43.84 48.84,44.48 48.84,44.94 49.69,45.79 50.59,45.79 51.36,45.02 v51.36,44.74 51.36,43.27 51.64,42.99 IC1.15
  Top 0.305: IC3.32 45.27,42.31 R18.1
  Bottom 0.254: TP4.TP 52.11,44.76 51.17,44.76 51.18,44.74 v51.36,44.74
VCC
  Top 0.406: IC1.1 62.75,35.06 66.3,31.51 J1.9

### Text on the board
tPlace: ADE9153A TEST BOARD | OUT | PHASE | IN | CT | NEUTRAL | CT | PWR | IBMS | CF2 | CF1 | IRQ | DANGER | DO NOT TOUCH | HIGH VOLTAGE
bPlace: CF2 | IRQ | RESET | SS | MISO | MOSI | CLK | GND | VCC | ADE9153A TEST BOARD | ENERGY METERING | V1.1 | Designed By: NK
